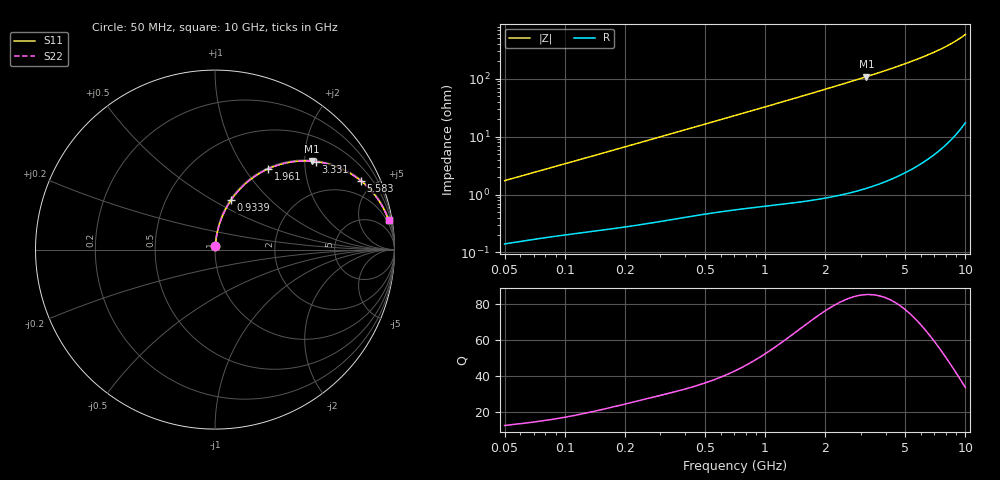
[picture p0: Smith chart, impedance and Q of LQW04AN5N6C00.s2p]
!Murata Part Number: LQW04AN5N6C00
!These Parameters are Measured in Series Mode Connection
!  o--[Z]--o
!Port1  Port2
!  o-------o
!Freq. Start=50[MHz] Stop=10[GHz], 401[Steps]
# Hz S RI R 50
!Freq.(Hz)	S 11(Real)	S 11(Imag)	S 21(Real)	S 21(Imag)	S 12(Real)	S 12(Imag)	S 22(Real)	S 22(Imag)
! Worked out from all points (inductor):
!   401 points, 50 MHz to 10 GHz, reference 50 ohm
!   read as one part in series: L = 5.47 nH near 51.34 MHz
!   highest Q = 85 at 3.201 GHz (marker M1), where L = 5.4 nH
!   S11 on the Smith chart (normalised r, x): 50 MHz: 1.00, +0.03; 933.9 MHz: 1.01, +0.61; 1.961 GHz: 1.02, +1.29; 3.331 GHz: 1.03, +2.27; 5.583 GHz: 1.06, +4.20; 10 GHz: 1, +12
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5e7  0.0017 0.0173  0.9983 -0.0173  0.9983 -0.0173  0.0017 0.0173
1.214486e8  0.00384 0.0407  0.9962 -0.0407  0.9962 -0.0407  0.00384 0.0407
1.956524e8  0.00693 0.0647  0.9931 -0.0647  0.9931 -0.0647  0.00693 0.0647
2.949953e8  0.0128 0.0962  0.9872 -0.0962  0.9872 -0.0962  0.0128 0.0962
4.628099e8  0.0268 0.1477  0.9732 -0.1477  0.9732 -0.1477  0.0268 0.1477
7.071068e8  0.0555 0.2176  0.9445 -0.2176  0.9445 -0.2176  0.0555 0.2176
9.338757e8  0.09 0.2763  0.91 -0.2763  0.91 -0.2763  0.09 0.2763
1.283367e9  0.1542 0.353  0.8458 -0.353  0.8458 -0.353  0.1542 0.353
1.484667e9  0.1954 0.389  0.8046 -0.389  0.8046 -0.389  0.1954 0.389
1.717543e9  0.245 0.4231  0.755 -0.4231  0.755 -0.4231  0.245 0.4231
1.9608e9  0.2977 0.4507  0.7023 -0.4507  0.7023 -0.4507  0.2977 0.4507
2.521925e9  0.4155 0.4868  0.5845 -0.4868  0.5845 -0.4868  0.4155 0.4868
3.200947e9  0.5411 0.4925  0.4589 -0.4925  0.4589 -0.4925  0.5411 0.4925
3.330706e9  0.5624 0.4902  0.4376 -0.4902  0.4376 -0.4902  0.5624 0.4902
4.171863e9  0.6801 0.4604  0.3199 -0.4604  0.3199 -0.4604  0.6801 0.4604
4.826234e9  0.7498 0.4268  0.2502 -0.4268  0.2502 -0.4268  0.7498 0.4268
5.583245e9  0.8117 0.3841  0.1883 -0.3841  0.1883 -0.3841  0.8117 0.3841
6.632392e9  0.8731 0.3249  0.1269 -0.3249  0.1269 -0.3249  0.8731 0.3249
7.672705e9  0.9146 0.2701  0.0854 -0.2701  0.0854 -0.2701  0.9146 0.2701
8.644138e9  0.9417 0.2233  0.0583 -0.2233  0.0583 -0.2233  0.9417 0.2233
9.738562e9  0.9629 0.1755  0.0371 -0.1755  0.0371 -0.1755  0.9629 0.1755
1e10  0.9668 0.1648  0.0332 -0.1648  0.0332 -0.1648  0.9668 0.1648
